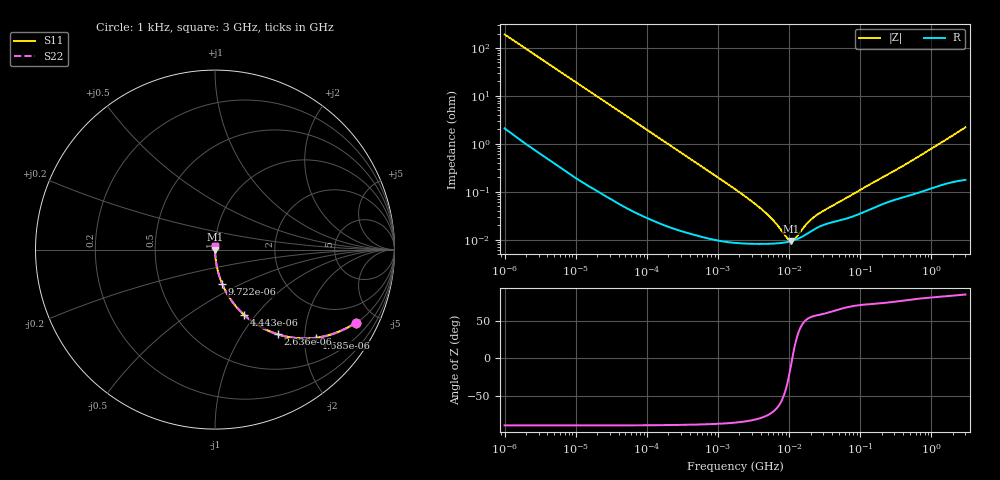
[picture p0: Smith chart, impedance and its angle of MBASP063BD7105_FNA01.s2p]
! MBASP063BD7105_FNA01  S-PARAMETER MODEL  ( Standard Model )
! Model Generated by TAIYO YUDEN Corporation (http://www.ty-top.com)
! Version 1.0
! TAIYO YUDEN Control No. 241206
! Copyright(c) 2024 TAIYO YUDEN CO.,LTD. All Rights Reserved.
! Product Description (link to TY-COMPAS)
! https://ds.yuden.co.jp/TYCOMPAS/or/detail?pn=MBASP063BD7105MFNA01&u=M
! Products Name : Multilayer Ceramic Capacitors
! Characteristics :
!  Capacitance : 1 [uF] , Rated Voltage : 2.5 [V] , TCC : X7T
!  Case Size : 0.6 x 0.3 / 0.024 x 0.012 [mm/inch] , Thickness : 0.3 / 0.012 [mm/inch]
!  (Conditions: Temperature = 25 [degC] , DC Bias Voltage = 0 [V])
! External Node Assignments :
!  1  o---| |---o  2
! GND o---------o GND
! Frequency Range : 1kHz  -  3GHz  [ 401 STEP ]
# MHZ S RI R 50
! Freq[MHz].  S11 Real  S11 Imag  S21 Real  S21 Imag  S12 Real  S12 Imag  S22 Real  S22 Imag
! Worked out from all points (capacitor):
!   401 points, 1 kHz to 3 GHz, reference 50 ohm
!   read as one part in series: C = 830 nF near 1.077 kHz
!   lowest |Z| = 9.41 mohm at 10.76 MHz (marker M1)
!   series resonance near 11.05 MHz, so ESL is about 250 pH
!   S11 on the Smith chart (normalised r, x): 1 kHz: 1.04, -3.83; 1.685 kHz: 1.02, -2.28; 2.636 kHz: 1.01, -1.46; 4.443 kHz: 1.01, -0.87; 9.722 kHz: 1.00, -0.40; 3 GHz: 1.00, +0.04
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0.001  0.7828 -0.4069  0.2172 0.4069  0.2172 0.4069  0.7828 -0.4069
0.001251  0.6992 -0.4532  0.3008 0.4532  0.3008 0.4532  0.6992 -0.4532
0.001685  0.5641 -0.4907  0.4359 0.4907  0.4359 0.4907  0.5641 -0.4907
0.002636  0.3492 -0.4717  0.6508 0.4717  0.6508 0.4717  0.3492 -0.4717
0.004443  0.1614 -0.3629  0.8386 0.3629  0.8386 0.3629  0.1614 -0.3629
0.006451  0.0849 -0.2738  0.9151 0.2738  0.9151 0.2738  0.0849 -0.2738
0.009722  0.0401 -0.1912  0.9599 0.1912  0.9599 0.1912  0.0401 -0.1912
0.01216  0.0264 -0.1553  0.9736 0.1553  0.9736 0.1553  0.0264 -0.1553
0.033275  0.00409 -0.0585  0.9959 0.0585  0.9959 0.0585  0.00409 -0.0585
0.147855  0.000399 -0.0133  0.9996 0.0133  0.9996 0.0133  0.000399 -0.0133
1.732051  8.71e-05 -0.00113  0.9999 0.00113  0.9999 0.00113  8.71e-05 -0.00113
3.03007  8.24e-05 -0.000615  0.9999 0.000615  0.9999 0.000615  8.24e-05 -0.000615
4.566395  8.19e-05 -0.000367  0.9999 0.000367  0.9999 0.000367  8.19e-05 -0.000367
6.387174  8.34e-05 -0.000211  0.9999 0.000211  0.9999 0.000211  8.34e-05 -0.000211
9.273352  8.9e-05 -6.47e-05  0.9999 6.47e-05  0.9999 6.47e-05  8.9e-05 -6.47e-05
10.76485  9.36e-05 -9.57e-06  0.9999 9.57e-06  0.9999 9.57e-06  9.36e-05 -9.57e-06
12.49624  0.000101 4.5e-05  0.9999 -4.5e-05  0.9999 -4.5e-05  0.000101 4.5e-05
16.83921  0.000126 0.000153  0.9999 -0.000153  0.9999 -0.000153  0.000126 0.000153
21.06097  0.000155 0.000229  0.9998 -0.000229  0.9998 -0.000229  0.000155 0.000229
29.45871  0.0002 0.000337  0.9998 -0.000337  0.9998 -0.000337  0.0002 0.000337
256.0921  0.000628 0.00231  0.9994 -0.00231  0.9994 -0.00231  0.000628 0.00231
3000  0.00225 0.0219  0.9978 -0.0219  0.9978 -0.0219  0.00225 0.0219
